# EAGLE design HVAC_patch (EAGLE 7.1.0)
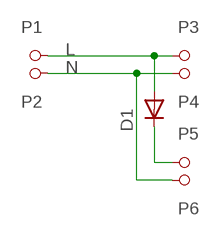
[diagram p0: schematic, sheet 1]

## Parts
D1  1N4148  DIODE-5MM  [DIODE-5MM]
P1  SPADE-3MM  [SPADE-3MM]
P2  SPADE-3MM  [SPADE-3MM]
P3  SPADE-3MM  [SPADE-3MM]
P4  SPADE-3MM  [SPADE-3MM]
P5  SPADE-3MM  [SPADE-3MM]
P6  SPADE-3MM  [SPADE-3MM]

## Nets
L: D1.A P1.P$1 P1.P$2 P3.P$1 P3.P$2
N: P2.P$1 P2.P$2 P4.P$1 P4.P$2 P6.P$1 P6.P$2
N$3: D1.C P5.P$1 P5.P$2

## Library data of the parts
D1 = 1Axel:DIODE-5MM: Diode 5mm
P1-P6 = Axel:SPADE-3MM

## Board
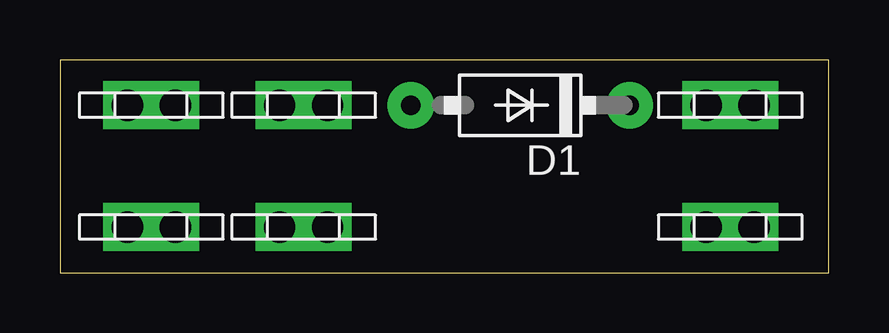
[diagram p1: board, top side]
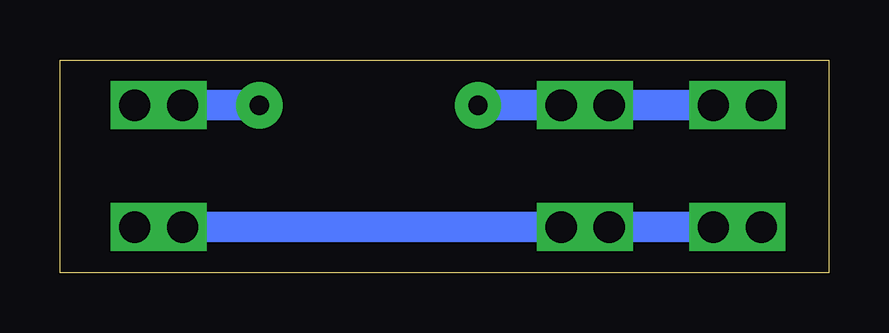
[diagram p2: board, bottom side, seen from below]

Size 32.05 x 8.88 mm. Coordinates in mm from the lower left corner, seen from the top.
Outline: 0,0 32.05,0 32.05,8.88 0,8.88 0,0
Copper layers (1*16): Top 0.035mm / dielectric 1.5mm / Bottom 0.035mm
Design rules "default": minimum track width 10mil, minimum drill 24mil, track to track 8mil, track to pad 8mil, pad to pad 8mil, via to via 8mil, smd to smd 8mil, copper to edge 40mil, drill to drill 8mil, minimum pad ring 10mil, minimum via ring 8mil, stop-mask expansion 4mil, vias tented up to drill 0mil, thermal gap 10mil

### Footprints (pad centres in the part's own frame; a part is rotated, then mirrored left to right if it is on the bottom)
DIODE-5MM = drill 0.8 pad 1.93: A 5.06,0; C -4.06,0
SPADE-3MM = drill 1.3 pad 2 square: P$1 0,1; P$2 0,-1

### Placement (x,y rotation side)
D1  19.68,6.99 180 top
P1  3.81,6.99 90 top
P2  10.16,1.91 90 top
P3  10.16,6.99 90 top
P4  3.81,1.91 90 top
P5  27.94,6.99 90 top
P6  27.94,1.91 90 top

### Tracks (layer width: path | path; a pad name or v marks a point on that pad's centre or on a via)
L
  Bottom 1.016: P1.P$1 P1.P$2
  Bottom 1.27: P1.P$1 P3.P$1 P3.P$2 D1.A
N
  Bottom 1.27: P4.P$1 P4.P$2 P2.P$1 P2.P$2 P6.P$1 P6.P$2
N$3
  Bottom 1.27: D1.C P5.P$1 P5.P$2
